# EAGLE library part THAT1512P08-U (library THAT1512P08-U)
THAT CORPORATION - THAT1512P08-U - IC, PRE-AMP, MICROPHONE, DIP8 Source: Datasheet
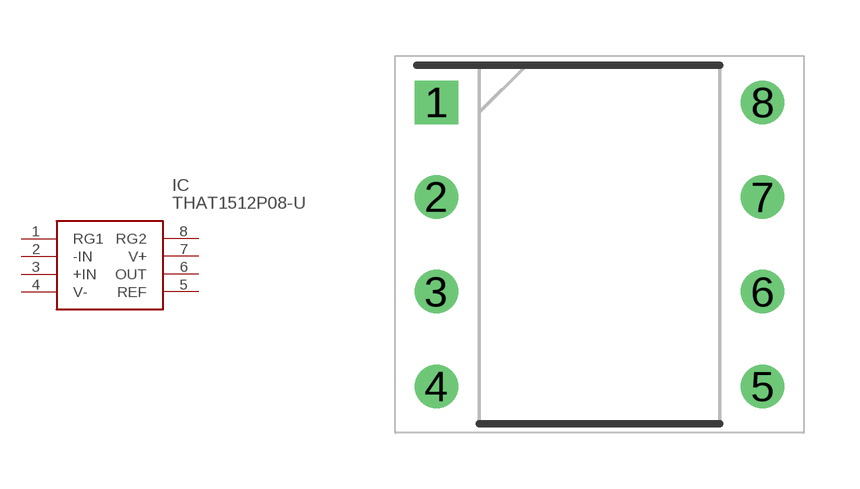
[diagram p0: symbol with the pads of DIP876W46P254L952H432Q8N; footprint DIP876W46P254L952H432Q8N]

Designator prefix IC

## THAT1512P08-U (Description: THAT CORPORATION - THAT1512P08-U - IC, PRE-AMP, MICROPHONE, DIP8; Height: 4.32mm; Manufacturer_Name: THAT CORPORATION; Manufacturer_Part_Number: THAT1512P08-U)  [DIP876W46P254L952H432Q8N]
1  RG1
2  -IN  in
3  +IN  in
4  V-  pwr
5  REF  pwr
6  OUT  out
7  V+  pwr
8  RG2

## Footprint DIP876W46P254L952H432Q8N (pad centres in mm)
1512
drill 0.66 pad 1.06 square: 1 -4.382,3.81
drill 0.66 pad 1.06: 2 -4.382,1.27; 3 -4.382,-1.27; 4 -4.382,-3.81; 5 4.382,-3.81; 6 4.382,-1.27; 7 4.382,1.27; 8 4.382,3.81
